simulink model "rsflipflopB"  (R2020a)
settings: Solver=ode45  StartTime=0.0  StopTime=Inf  FixedStep=1  RelTol=1e-3  EnableMultiTasking=on

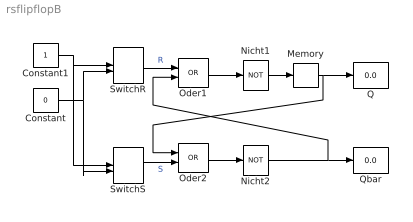
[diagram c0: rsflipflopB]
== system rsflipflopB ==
  Constant : Constant  Value=0
  Constant1 : Constant
  Memory : Memory  LinearizeMemory=on
  Nicht1 : Logic  Operator=NOT  AllPortsSameDT=off
  Nicht2 : Logic  Operator=NOT  AllPortsSameDT=off
  Oder1 : Logic  Operator=OR  AllPortsSameDT=off
  Oder2 : Logic  Operator=OR  AllPortsSameDT=off
  Q : Display
  Qbar : Display
  SwitchR : ManualSwitch  CurrentSetting=0
  SwitchS : ManualSwitch  CurrentSetting=0
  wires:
  Oder2/1 -> Nicht2/1
  Nicht1/1 -> Memory/1
  Nicht2/1 -> Oder1/2, Qbar/1
  SwitchR/1 -> Oder1/1  "R"
  Constant1/1 -> SwitchS/1, SwitchR/1
  Constant/1 -> SwitchS/2, SwitchR/2
  SwitchS/1 -> Oder2/2  "S"
  Oder1/1 -> Nicht1/1
  Memory/1 -> Oder2/1, Q/1
